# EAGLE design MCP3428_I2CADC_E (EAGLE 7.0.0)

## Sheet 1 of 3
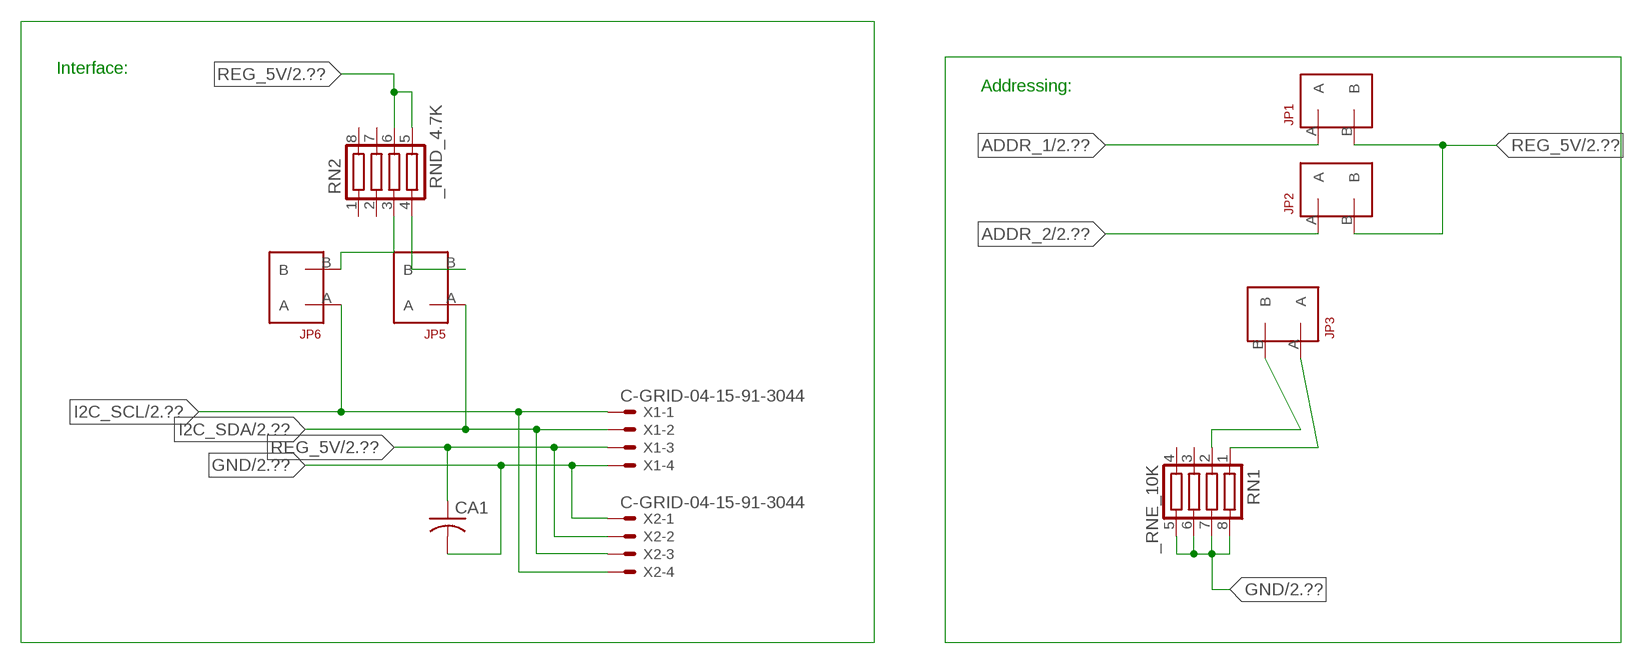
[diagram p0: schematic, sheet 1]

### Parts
CA1  CC1206KRX7R9BB104  [.1UF]
JP1  JUMPER_1X2_2MM  [JUMPER_1X2_2MM]
JP2  JUMPER_1X2_2MM  [JUMPER_1X2_2MM]
JP3  JUMPER_1X2_2MM  [JUMPER_1X2_2MM]
JP5  JUMPER_1X2_2MM  [JUMPER_1X2_2MM]
JP6  JUMPER_1X2_2MM  [JUMPER_1X2_2MM]
RN1  _RNE_10K  [RNE]
RN2  _RND_4.7K  [RND]
X1  C-GRID-04-15-91-3044  [15-91-04]
X2  C-GRID-04-15-91-3044  [15-91-04]

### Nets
ADDR_1: JP1.A ; also sheet 2
ADDR_2: JP2.A ; also sheet 2
GND: CA1.2 RN1.5 RN1.6 RN1.7 RN1.8 X1.4 X2.1 ; also sheet 2,3
I2C_SCL: JP6.A X1.1 X2.4 ; also sheet 2
I2C_SDA: JP5.A X1.2 X2.3 ; also sheet 2
N$1: JP6.B RN2.3
N$2: JP5.B RN2.4
N$3: JP3.A RN1.1
N$5: JP3.B RN1.2
REG_5V: CA1.1 JP1.B JP2.B RN2.5 RN2.6 X1.3 X2.2 ; also sheet 2,3
Unconnected: RN1.3 RN1.4 RN2.1 RN2.2 RN2.7 RN2.8

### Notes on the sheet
- Interface:
- Addressing:

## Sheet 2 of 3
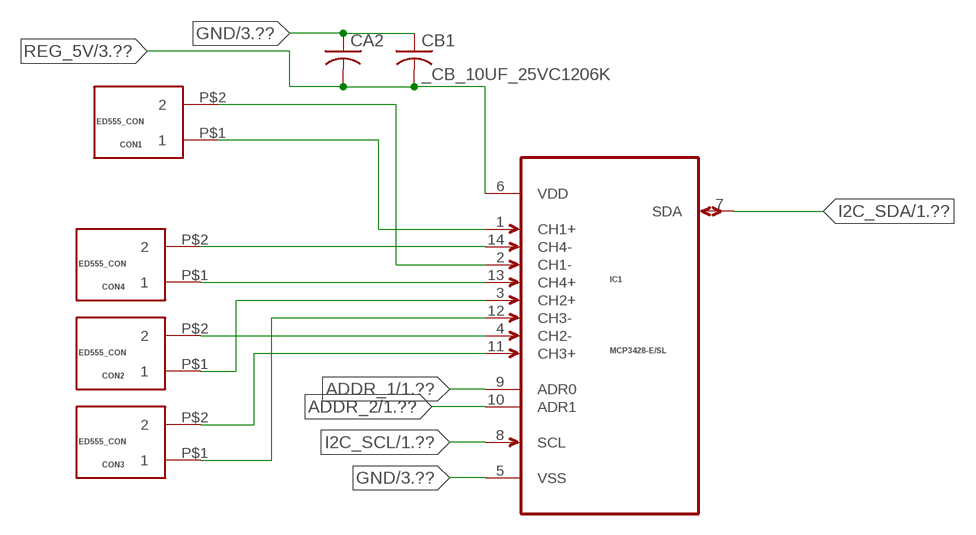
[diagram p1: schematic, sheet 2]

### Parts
CA2  _CA_.10UF_50VC1206K  [_CA_.1UF_50V]
CB1  _CB_10UF_25VC1206K  [_CB_10UF_25V]
CON1  ED555_CON  [ED555_CON]
CON2  ED555_CON  [ED555_CON]
CON3  ED555_CON  [ED555_CON]
CON4  ED555_CON  [ED555_CON]
IC1  MCP3428-E/SL  [SOIC127P600X175-14N]

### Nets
ADDR_1: IC1.9(ADR0) ; also sheet 1
ADDR_2: IC1.10(ADR1) ; also sheet 1
GND: CA2.1 CB1.1 IC1.5(VSS) ; also sheet 1,3
I2C_SCL: IC1.8(SCL) ; also sheet 1
I2C_SDA: IC1.7(SDA) ; also sheet 1
N$6: CON1.P$2 IC1.2(CH1-)
N$7: CON1.P$1 IC1.1(CH1+)
N$8: CON2.P$1 IC1.3(CH2+)
N$9: CON2.P$2 IC1.4(CH2-)
N$10: CON4.P$2 IC1.14(CH4-)
N$11: CON4.P$1 IC1.13(CH4+)
N$12: CON3.P$2 IC1.11(CH3+)
N$13: CON3.P$1 IC1.12(CH3-)
REG_5V: CA2.2 CB1.2 IC1.6(VDD) ; also sheet 1,3

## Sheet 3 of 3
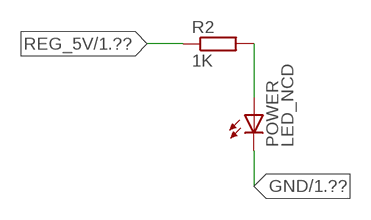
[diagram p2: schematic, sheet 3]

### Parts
POWER  LED_NCD  [CHIPLED_0603]
R2  1K  RESISTOR_SMT-0402  [R402]

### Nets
GND: POWER.C ; also sheet 1,2
N$23: POWER.A R2.2
REG_5V: R2.1 ; also sheet 1,2

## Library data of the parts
CA1 = NCD_ULTIMATE_LIBRARY:CC1206KRX7R9BB104: Capacitor CA .1uF 50V SMT C1206K CC1206KRX7R9BB104
CA2 = NCD_ULTIMATE_LIBRARY:_CA_.10UF_50V: Capacitor .1uF SMT
CB1 = NCD_ULTIMATE_LIBRARY:_CB_10UF_25V: Capacitor 10uF SMT
CON1-CON4 = NCD_ULTIMATE_bhaskar:ED555_CON: Digikey ED1514-ND/ ED555/2DS NCD CON
IC1 = NCD_ULTIMATE_bhaskar:MCP3428-E/SL: Digikey MCP3428-E/SL-ND/ MCP3428-E/SL; MPN: MCP3428-E/SL; OC_FARNELL: 1825014; OC_NEWARK: 52R9962; PACKAGE: SOIC-14; SUPPLIER: Microchip
JP1-JP3 JP5 JP6 = NCD_ULTIMATE_CONNECTORS:JUMPER_1X2_2MM
POWER = NCD_ULTIMATE_LIBRARY:LED_NCD: LED Digikey 754-1132-2-ND/APT2012SRCPRV
R2 = NCD_ULTIMATE_LIBRARY:RESISTOR_SMT: NCD Resistor
RN1 = NCD_ULTIMATE_LIBRARY:_RNE_10K: Resistor Array RNE SMT 10K x 4 Single Resistor Source: http://www.ctscorp.com/components/Datasheets/CTSChipArrayDs.pdf Digikey 742C083103JPTR-ND/742C083103JP; OC_FARNELL: unknown; OC_NEWARK: unknown
RN2 = NCD_ULTIMATE_LIBRARY:_RND_4.7K: Resistor Array RND SMT 4.7K x 4 Single Resistor Source: http://www.ctscorp.com/components/Datasheets/CTSChipArrayDs.pdf Digikey 742C083472JPTR-ND/742C083472JP; OC_FARNELL: unknown; OC_NEWARK: unknown
X1 X2 = NCD_ULTIMATE_CONNECTORS:C-GRID-04: CONNECTOR 4-Pos I2C wire to board 2.54 mm (0.100") pitch header Digikey WM1342-ND/0015912045; OC_FARNELL: unknown; OC_NEWARK: unknown

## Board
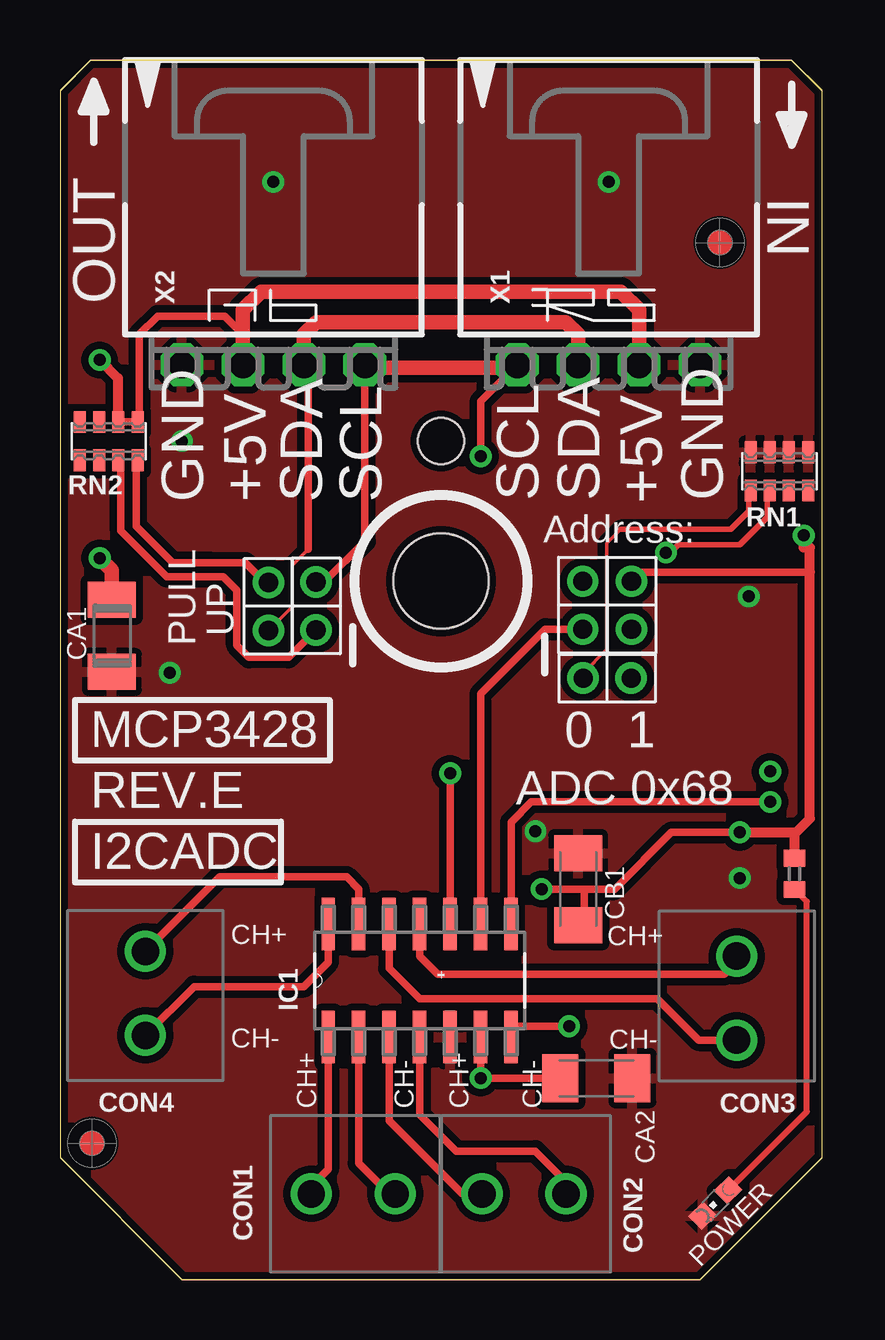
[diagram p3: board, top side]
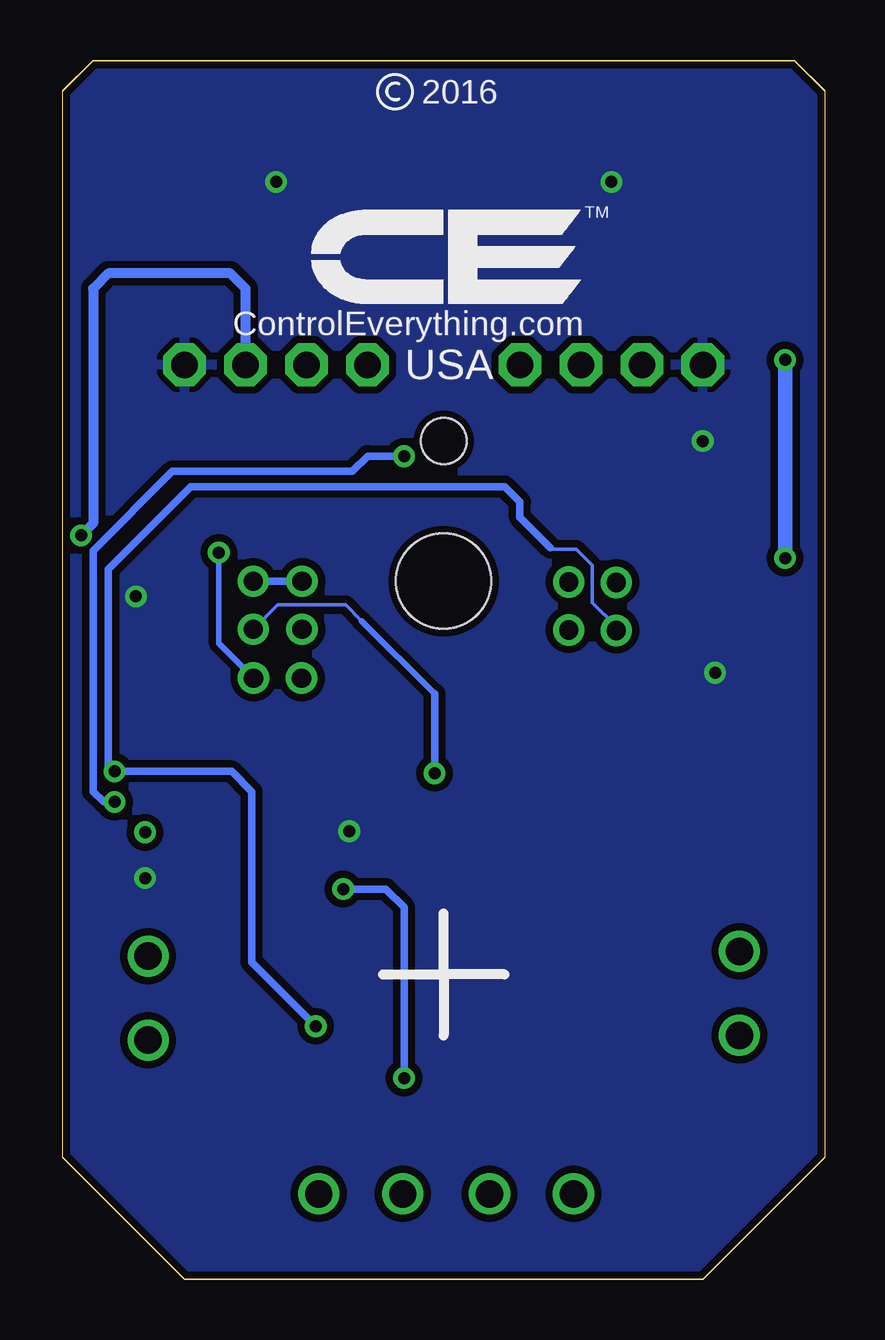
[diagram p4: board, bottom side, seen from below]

Size 31.75 x 50.83 mm. Coordinates in mm from the lower left corner, seen from the top.
Outline: 31.75,5.08 31.75,49.53 30.48,50.8 1.27,50.8 0,49.53 0,5.08 5.08,0 26.67,0 31.75,5.08
Outline: 31.75,5.11 31.75,49.56 30.48,50.83 1.27,50.83 0,49.56 0,5.11 5.08,0.03 26.67,0.03 31.75,5.11
Outline: 31.75,5.11 31.75,49.56 30.48,50.83 1.27,50.83 0,49.56 0,5.11 5.08,0.03 26.67,0.03 31.75,5.11
Copper layers (1*16): Top 0.035mm / dielectric 1.5mm / Bottom 0.035mm
Design rules "default": minimum track width 5mil, minimum drill 24mil, track to track 5mil, track to pad 5mil, pad to pad 5mil, via to via 5mil, smd to smd 5mil, copper to edge 10mil, drill to drill 8mil, minimum pad ring 10mil, minimum via ring 8mil, stop-mask expansion 2mil, vias tented up to drill 0mil, thermal gap 10mil
Holes 3.96 mm at 15.88,29.11
Holes 1.91 mm at 15.88,34.95

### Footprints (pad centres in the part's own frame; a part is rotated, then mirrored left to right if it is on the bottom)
.1UF = smd 1.5 x 2: 1 -1.5,0; 2 1.5,0
_CA_.1UF_50V = smd 1.5 x 2: 1 -1.5,0; 2 1.5,0
_CB_10UF_25V = smd 1.5 x 2: 1 -1.5,0; 2 1.5,0
ED555_CON = drill 1.143: P$1 0,3.5; P$2 0,0
SOIC127P600X175-14N = smd 2.184 x 0.559: 1 -2.362,3.81; 2 -2.362,2.54; 3 -2.362,1.27; 4 -2.362,0; 5 -2.362,-1.27; 6 -2.362,-2.54; 7 -2.362,-3.81; 8 2.362,-3.81; 9 2.362,-2.54; 10 2.362,-1.27; 11 2.362,0; 12 2.362,1.27; 13 2.362,2.54; 14 2.362,3.81
JUMPER_1X2_2MM = drill 0.8: A 0,2; B 0,0
CHIPLED_0603 = smd 0.8 x 0.876: A 0,-0.75; C 0,0.75
R402 = smd 0.7 x 0.9: 1 -0.65,0; 2 0.65,0
RNE = smd 0.5 x 0.9: 1 -1.2,-0.8; 2 -0.4,-0.8; 3 0.4,-0.8; 4 1.2,-0.8; 5 1.2,0.8; 6 0.4,0.8; 7 -0.4,0.8; 8 -1.2,0.8
RND = smd 0.5 x 0.9: 1 -1.2,-0.8; 2 -0.4,-0.8; 3 0.4,-0.8; 4 1.2,-0.8; 5 1.2,0.8; 6 0.4,0.8; 7 -0.4,0.8; 8 -1.2,0.8
15-91-04 = drill 1.1 pad 1.778 octagon: 1 -3.81,-7.62; 2 -1.27,-7.62; 3 1.27,-7.62; 4 3.81,-7.62

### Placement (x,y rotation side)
CA1  2.16,26.84 270 top
CA2  22.35,8.41 180 top
CB1  21.59,16.28 270 top
CON1  13.97,3.58 90 top
CON2  21.08,3.58 90 top
CON3  28.19,13.49 180 top
CON4  3.56,10.19 0 top
IC1  14.99,12.47 90 top
JP1  21.78,29.11 180 top
JP2  23.81,29.11 180 top
JP3  23.8,25.07 90 top
JP5  8.69,29.06 180 top
JP6  10.67,27.08 0 top
POWER  27.3,3.2 135 top
R2  30.61,16.92 270 top
RN1  29.97,33.68 0 top
RN2  2.03,34.95 0 top
U$5  [VISION_REF10]  1.33,5.69 90 top
U$28  [VISION_REF10]  27.5,43.22 90 top
X1  22.86,45.75 0 top
X2  8.89,45.75 0 top

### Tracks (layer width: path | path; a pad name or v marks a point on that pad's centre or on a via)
ADDR_1
  Top 0.305: IC1.9 17.53,24.41 20.23,27.11 JP1.A
ADDR_2  (via drill 0.5)
  Top 0.305: IC1.10 v16.26,21.11
  Bottom 0.152: 19.3,27.46 19.96,28.12 22.78,28.12 23.79,27.11 JP2.A
  Bottom 0.229: 16.26,24.41 19.3,27.46
  Bottom 0.305: v16.26,21.11 16.26,24.41
GND  (via drill 0.5)
  other vias: 8.89,45.75 22.86,45.75 28.32,16.74 4.57,25.3 28.7,28.47 5.08,34.95 19.81,18.69
  pour Bottom (isolate 0.305): 4.45,-0.61 -0.64,4.47 -0.64,50.19 0.64,51.46 31.11,51.46 32.38,50.19 32.38,4.47 27.3,-0.61
  pour Top (isolate 0.305): 3.81,-1.24 -1.27,3.84 -1.27,50.83 0,52.1 31.75,52.1 33.02,50.83 33.02,3.84 27.94,-1.24
I2C_SCL  (via drill 0.5)
  Top 0.305: 12.7,38 12.7,30.76 11.02,29.08 JP6.A | v17.53,34.32 17.53,36.6 X1.1 | IC1.8 18.8,19.08 19.63,19.91 v29.59,19.91
  Top 0.406: X2.4 12.7,38 | 19.05,38 X1.1
  Top 0.61: 12.7,38 19.05,38
  Bottom 0.305: v29.59,19.91 30.05,19.91 30.48,20.35 30.48,30.38 27.18,33.68 19.68,33.68 19.05,34.32 v17.53,34.32
I2C_SDA  (via drill 0.5)
  Top 0.152: 10.35,30.44 9.68,29.77 9.68,28.04 JP5.A
  Top 0.305: 10.35,30.44 10.35,37.93 X2.3 | IC1.7 18.8,10.69 18.92,10.57 v21.21,10.57
  Top 0.61: X2.3 10.16,39.4 10.67,39.9 21.08,39.9 21.59,39.4 X1.2
  Bottom 0.152: 11.43,30.51 11.37,30.44 10.35,30.44 9.68,29.77 9.68,28.22 8.69,27.23 JP5.A
  Bottom 0.305: 11.43,30.51 12.7,31.78 12.7,32.41 13.34,33.05 26.42,33.05 29.84,29.62 29.84,21.44 v29.59,21.18 24.71,21.18 23.88,20.35 23.88,13.23 v21.21,10.57
N$1
  Top 0.305: RN2.3 2.54,34.04 2.54,31.2 4.45,29.3 6.79,29.3 7.37,28.73 7.37,26.44 7.87,25.93 9.53,25.93 JP6.B
N$2
  Top 0.305: 6.35,29.87 4.7,29.87 3.17,31.39 3.17,34.09 RN2.4 | 6.35,29.87 | 6.35,29.87 7.72,29.87 8.53,29.06 JP5.B
N$3
  Top 0.152: 23.37,31.27 22.78,30.68 22.78,26.26 21.8,25.28 JP3.A
  Top 0.229: RN1.1 28.7,32.81 28.7,32.03 27.94,31.27 23.37,31.27
N$5  (via drill 0.5)
  Top 0.229: RN1.2 29.46,32.77 29.46,31.78 28.32,30.63 25.76,30.63 25.43,30.3 v25.25,30.3
  Bottom 0.229: 24.89,30.33 v25.25,30.3 25.25,26.52 JP3.B
N$6
  Top 0.305: IC1.2 12.45,4.85 13.72,3.58 CON1.P$2
N$7
  Top 0.305: IC1.1 11.18,4.6 10.47,3.89 CON1.P$1
N$8
  Top 0.305: IC1.3 13.72,6.63 16.76,3.58 CON2.P$1
N$9
  Top 0.305: IC1.4 14.99,6.88 16.51,5.36 19.81,5.36 21.08,4.09 CON2.P$2
N$10
  Top 0.305: CON4.P$2 5.59,12.22 10.16,12.22 11.18,13.23 IC1.14
N$11
  Top 0.305: CON4.P$1 6.66,16.79 11.94,16.79 12.45,16.28 IC1.13
N$12
  Top 0.305: IC1.11 14.99,13.49 15.75,12.73 27.69,12.73 28.19,13.23 CON3.P$2
N$13
  Top 0.305: IC1.12 13.72,12.98 14.99,11.71 24.89,11.71 26.61,9.99 CON3.P$1
N$23
  Top 0.254: POWER.A 31.11,7.01 31.11,15.76 R2.2
REG_5V  (via drill 0.5)
  Top 0.305: 7.62,39.4 7.49,39.4 | RN2.6 RN2.5 3.3,35.82 3.3,39.4 4.06,40.16 6.86,40.16 7.62,39.4 | X2.2 7.62,39.4 | CA2.2 17.78,8.41 17.53,8.66 IC1.6 v17.53,8.41 | v28.32,18.64 25.48,18.64 23.11,16.28 21.84,16.28 | CB1.2 21.84,15.52 21.84,16.28 | v20.07,16.28 21.84,16.28 | JP2.B 24.19,29.49 31.24,29.49
  Top 0.406: v28.32,18.64 30.48,18.64 | 30.48,18.64 30.67,18.64 31.24,19.22 31.24,29.49 31.24,30.51 30.99,30.51 v30.99,31.01 | v1.65,38.33 2.41,37.57 2.41,35.77 RN2.6 | R2.1 30.61,18.52 30.48,18.64
  Top 0.61: X1.3 24.13,40.41 23.37,41.17 8.38,41.17 7.62,40.41 X2.2 | CA1.1 2.16,29.57 v1.65,30.07
  Top 0.813: v30.99,31.01 31.05,31.01
  Bottom 0.305: v17.53,8.41 17.53,15.52 18.29,16.28 v20.07,16.28 | JP1.B JP2.B
  Bottom 0.406: X1.3 24.13,41.3 24.77,41.94 29.84,41.94 30.48,41.3 30.48,31.52 v30.99,31.01
  Bottom 0.61: v1.65,30.07 v1.65,38.33

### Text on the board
tPlace: CH+ | CH+ | CH- | CH- | CH+ | CH- | CH+ | CH-
tNames: IN | OUT | GND | +5V | SDA | SCL | SCL | SDA | +5V | GND | Address: | UP | PULL | MCP3428 | 0 | 1 | ADC 0x68 | REV.E | I2CADC
bNames: 2016 | TM | ControlEverything.com | USA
